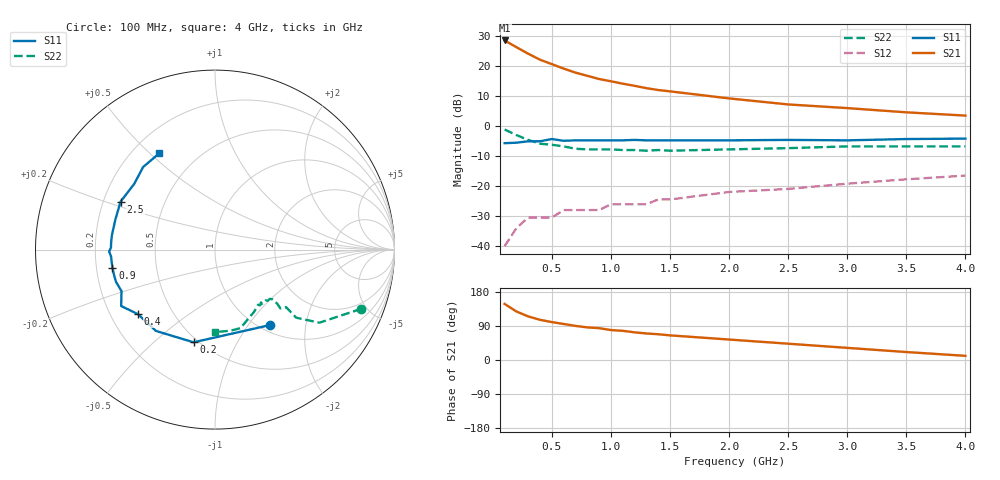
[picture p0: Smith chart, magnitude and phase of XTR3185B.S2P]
! HXTR-3185
! Typical S-Parameters Vce = 10 V, Ic = 15 mA
# ghz s ma r 50
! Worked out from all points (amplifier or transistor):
!   20 points, 100 MHz to 4 GHz, reference 50 ohm
!   highest |S21| = 28.6 dB at 100 MHz (marker M1)
!   |S21| within 3 dB of that: start of sweep to 234.7 MHz
!   unconditionally stable (mu >= 1): 881.6 MHz to 915.8 MHz; 1.116 GHz to 3.289 GHz
!   at 400 MHz: K = 0.60, MSG = 26.3 dB, |S12| = -30.5 dB
!   at 1.1 GHz: K = 0.99, MSG = 20.1 dB, |S12| = -26.0 dB
!   at 4 GHz: K = 0.95, MSG = 10.0 dB, |S12| = -16.5 dB
!   S11 on the Smith chart (normalised r, x): 100 MHz: 1.11, -1.28; 200 MHz: 0.47, -0.68; 400 MHz: 0.32, -0.33; 900 MHz: 0.27, -0.08; 2.5 GHz: 0.27, +0.22; 4 GHz: 0.31, +0.54
0.1  0.52 -54.0  26.8 148.0  0.01 66.0  0.88 -22.0
0.2  0.53 -103.0  20.7 128.0  0.02 53.0  0.71 -35.0
0.3  0.56 -126.0  16.1 115.0  0.03 48.0  0.59 -40.0
0.4  0.56 -140.0  12.8 106.0  0.03 47.0  0.51 -39.0
0.5  0.61 -149.0  10.8 100.0  0.03 47.0  0.49 -42.0
0.6  0.57 -156.0  9.1 95.0  0.04 47.0  0.46 -41.0
0.7  0.58 -162.0  7.8 90.0  0.04 48.0  0.42 -41.0
0.8  0.58 -166.0  6.9 86.0  0.04 49.0  0.41 -42.0
0.9  0.58 -170.0  6.1 84.0  0.04 51.0  0.41 -42.0
1  0.58 -173.0  5.6 79.0  0.05 52.0  0.41 -44.0
1.1  0.58 -176.0  5.1 77.0  0.05 53.0  0.4 -45.0
1.2  0.59 -179.0  4.7 73.0  0.05 53.0  0.4 -49.0
1.3  0.58 179.0  4.3 70.0  0.05 54.0  0.39 -49.0
1.4  0.58 176.0  4 68.0  0.06 54.0  0.4 -51.0
1.5  0.58 172.0  3.8 65.0  0.06 55.0  0.39 -52.0
2  0.58 163.0  2.9 54.0  0.08 56.0  0.41 -58.0
2.5  0.59 153.0  2.3 43.0  0.09 56.0  0.43 -65.0
3  0.58 141.0  2 32.0  0.11 54.0  0.46 -72.0
3.5  0.61 131.0  1.7 21.0  0.13 52.0  0.46 -79.0
4  0.62 120.0  1.5 11.0  0.15 50.0  0.46 -90.0
